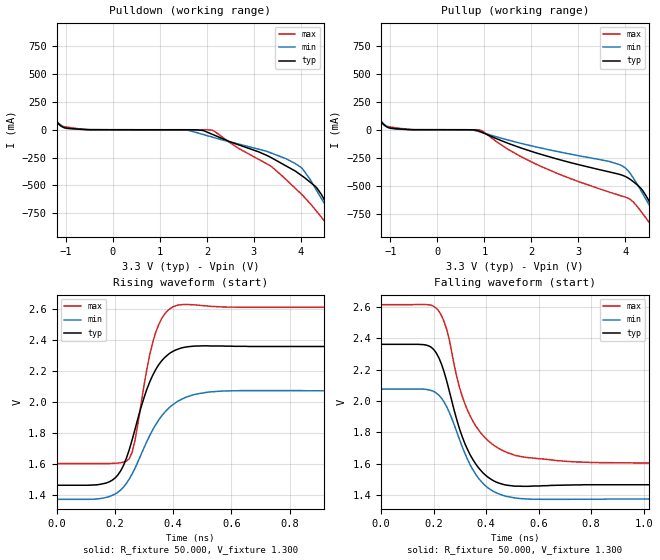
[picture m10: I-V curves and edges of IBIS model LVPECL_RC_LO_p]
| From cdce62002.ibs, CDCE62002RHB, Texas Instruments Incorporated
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|   Model LVPECL_RC_LO_p LVPECL LO SWING for UXP Pins
[Model]   LVPECL_RC_LO_p
Model_type   Output_ECL
Polarity   Non-Inverting
Enable   Active-High
Vmeas = 1.5
Vref = 0
Cref = 0
Rref = 150
|   typ   min   max
|   Strong PVT   Nominal PVT  Weak PVT
C_comp   1.8497pF   1.8465pF   1.8619pF
[Voltage Range]   3.3   3   3.6
[Temperature Range]   40   100   -40
[Pullup Reference]   3.3   3   3.6
[Pulldown Reference]   3.3   3   3.6
[Power Clamp Reference]   3.3   3   3.6
[GND Clamp Reference]   0   0   0
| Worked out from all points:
|   falling waveform, R_fixture 50.000, V_fixture 1.300: 20-80 % time 103ps typ, 110ps min, 118ps max; typ from 2.36 V to 1.47 V
|   rising waveform, R_fixture 50.000, V_fixture 1.300: 20-80 % time 91.4ps typ, 118ps min, 59.9ps max; typ from 1.47 V to 2.36 V
[Pulldown]
|   Voltage   I(typ)   I(min)   I(max)
-3.3V     1.332A     1.268A     1.424A
-2.68V    935.4mA    899.2mA    1.004A
-1.288V   115mA      119.3mA    116.2mA
-1.042V   18.84mA    20.53mA    27.56mA
1.586V    -109.5uA   -4.153mA   -17.03uA
2.111V    -40.58mA   -65.67mA   -4.131mA
3.352V    -247mA     -206.9mA   -324.1mA
3.992V    -405.1mA   -335.5mA   -571.5mA
4.342V    -525.1mA   -551.5mA   -737.5mA
4.689V    -781.1mA   -805.6mA   -932mA
4.89V     -953.1mA   -957.8mA   -1.114A
6.6V      -2.418A    -2.277A    -2.862A
[Pullup]
|   Voltage   I(typ)   I(min)   I(max)
-3.3V     1.332A     1.269A     1.435A
-2.63V    904.6mA    868.5mA    966.5mA
-1.29V    115.3mA    120.4mA    117.6mA
-1.067V   23.18mA    26.86mA    29.91mA
918mV     -17.48mA   -20.67mA   -4.542mA
2.059V    -201.7mA   -150.1mA   -300mA
3.672V    -378.5mA   -285.8mA   -559.7mA
4.02V     -422.7mA   -350mA     -605.8mA
4.317V    -519.2mA   -535mA     -722.3mA
4.665V    -763.2mA   -788.8mA   -915mA
4.838V    -904.1mA   -917.4mA   -1.054A
6.6V      -2.409A    -2.271A    -2.848A
[Ramp]
R_load = 50
|   typ   min   max
dV/dt_r   0.557474/9.12219e-11   0.420554/1.18318e-10   0.605849/5.99991e-11
dV/dt_f   0.557443/1.02721e-10   0.420514/1.10073e-10   0.605859/1.1832e-10
[Falling Waveform]
R_fixture = 50.000
V_fixture = 1.300
V_fixture_min = 1.000
V_fixture_max = 1.600
C_fixture = 0.000
|  time   V(typ)   V(min)   V(max)
0s        2.361V     2.075V     2.614V
170ps     2.357V     2.074V     2.615V
220ps     2.276V     2.037V     2.574V
250ps     2.128V     1.963V     2.457V
300ps     1.816V     1.749V     2.08V
350ps     1.625V     1.56V      1.87V
420ps     1.499V     1.431V     1.729V
510ps     1.456V     1.381V     1.653V
800ps     1.465V     1.373V     NA
1.7ns     1.465V     1.374V     1.605V
[Rising Waveform]
R_fixture = 50.000
V_fixture = 1.300
V_fixture_min = 1.000
V_fixture_max = 1.600
C_fixture = 0.000
|  time   V(typ)   V(min)   V(max)
0s        1.465V     1.374V     1.605V
180ps     1.486V     1.391V     1.605V
220ps     1.557V     1.434V     1.61V
250ps     1.696V     1.506V     1.637V
270ps     1.83V      1.577V     1.76V
310ps     2.084V     1.747V     2.213V
340ps     2.21V      1.854V     2.449V
410ps     2.339V     1.999V     2.624V
580ps     2.363V     2.074V     2.616V
1.7ns     2.361V     2.075V     2.614V
